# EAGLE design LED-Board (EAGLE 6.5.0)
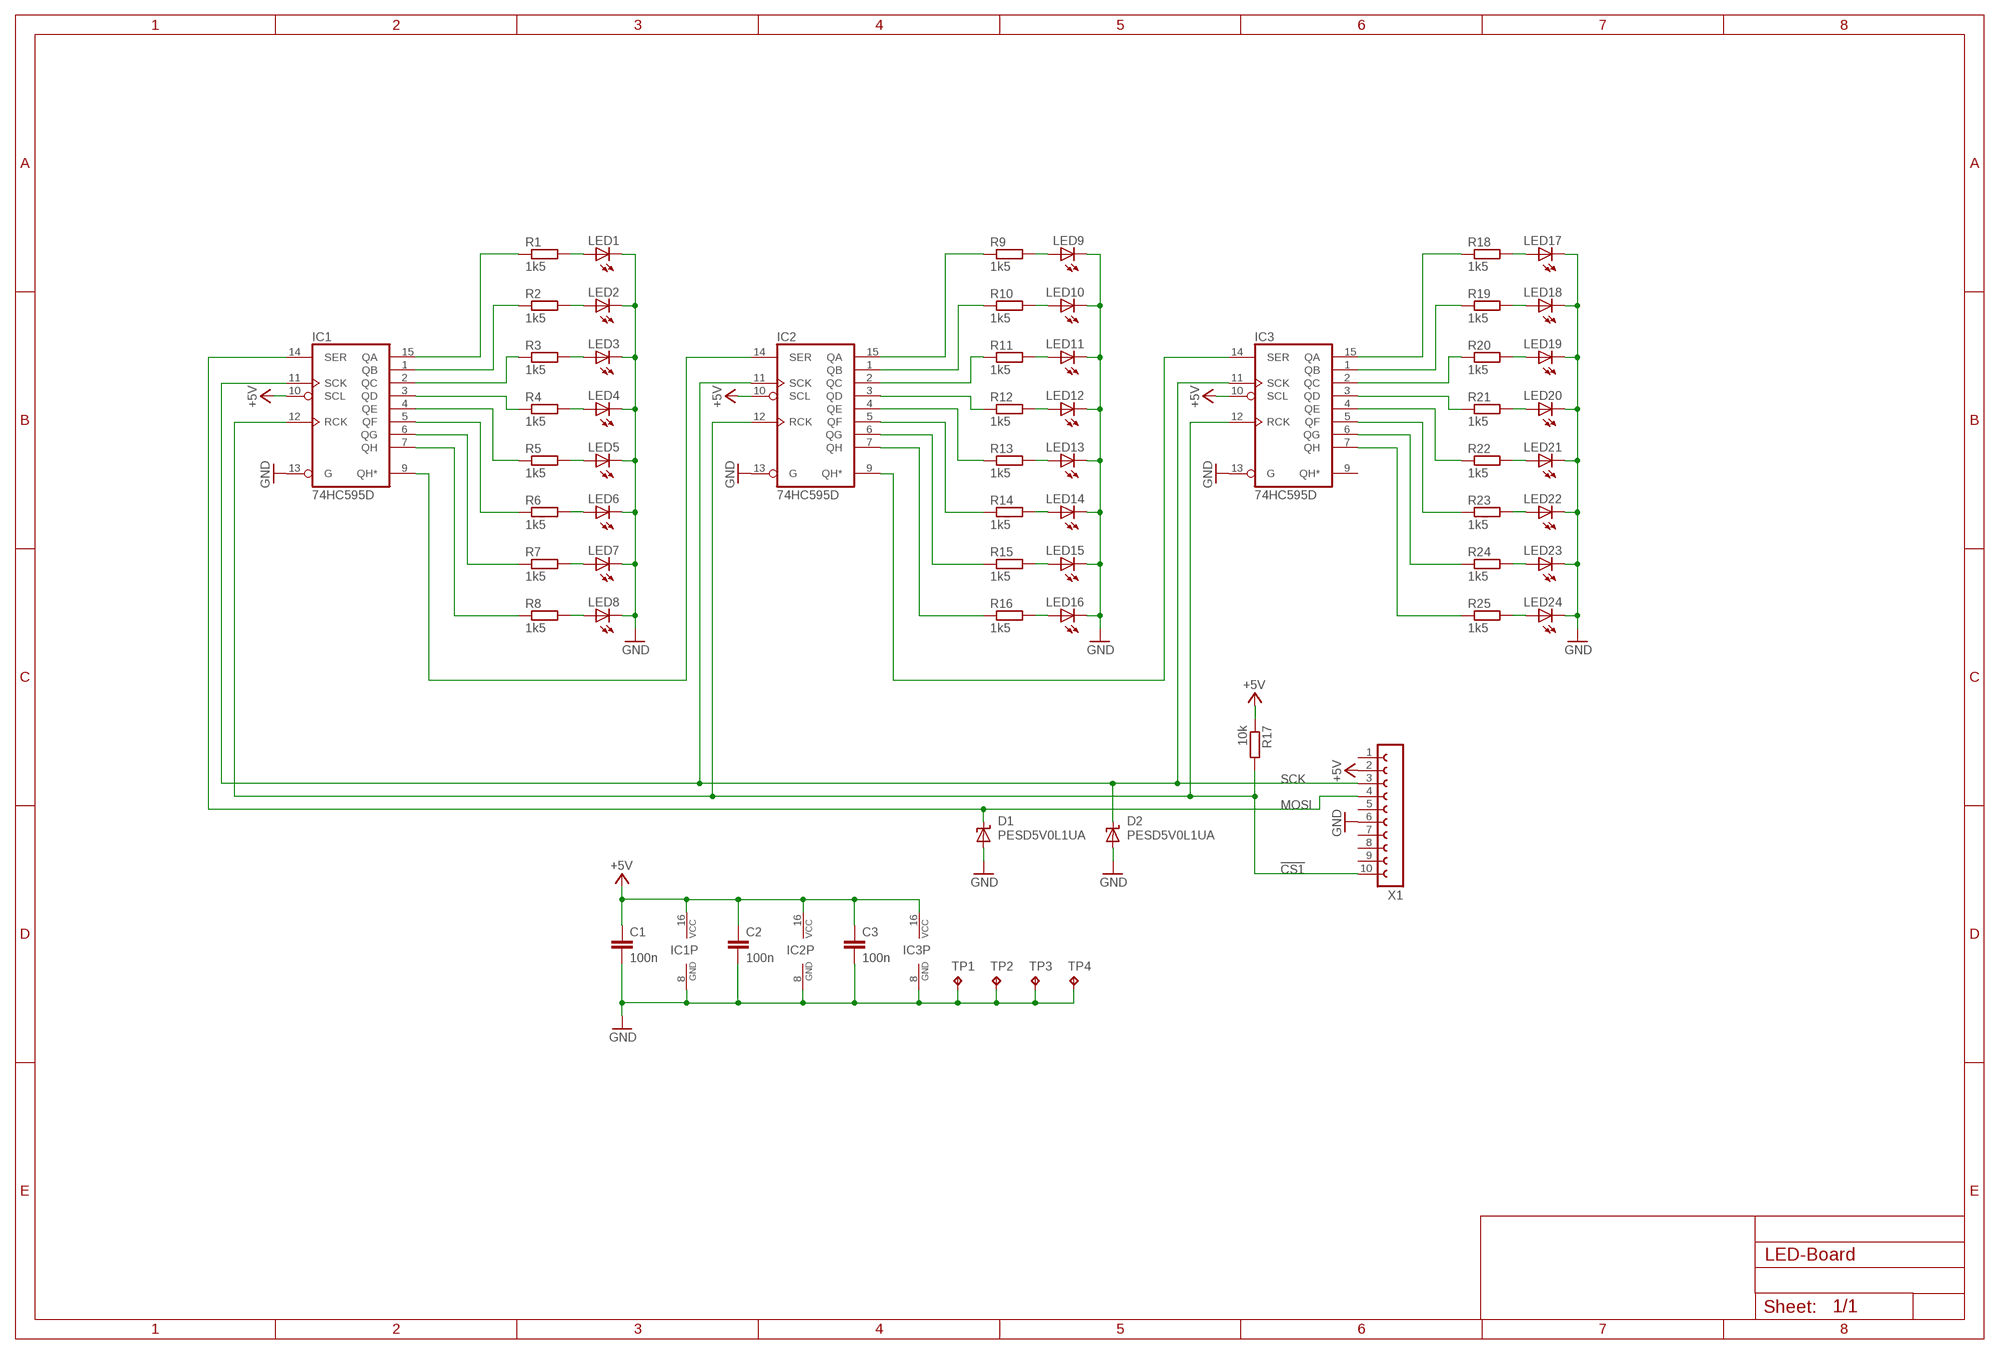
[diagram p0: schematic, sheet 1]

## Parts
C1  100n  C-EUC0603K  [C0603K]
C2  100n  C-EUC0603K  [C0603K]
C3  100n  C-EUC0603K  [C0603K]
D1  PESD5V0L1UA  SUPPRESSOR_UNI  [SOD323-W]
D2  PESD5V0L1UA  SUPPRESSOR_UNI  [SOD323-W]
IC1  74HC595D  [SO16]
IC2  74HC595D  [SO16]
IC3  74HC595D  [SO16]
LED1  LED3MM  [LED3MM]
LED2  LED3MM  [LED3MM]
LED3  LED3MM  [LED3MM]
LED4  LED3MM  [LED3MM]
LED5  LED3MM  [LED3MM]
LED6  LED3MM  [LED3MM]
LED7  LED3MM  [LED3MM]
LED8  LED3MM  [LED3MM]
LED9  LED3MM  [LED3MM]
LED10  LED3MM  [LED3MM]
LED11  LED3MM  [LED3MM]
LED12  LED3MM  [LED3MM]
LED13  LED3MM  [LED3MM]
LED14  LED3MM  [LED3MM]
LED15  LED3MM  [LED3MM]
LED16  LED3MM  [LED3MM]
LED17  LED3MM  [LED3MM]
LED18  LED3MM  [LED3MM]
LED19  LED3MM  [LED3MM]
LED20  LED3MM  [LED3MM]
LED21  LED3MM  [LED3MM]
LED22  LED3MM  [LED3MM]
LED23  LED3MM  [LED3MM]
LED24  LED3MM  [LED3MM]
R1  1k5  R-EU_R0603  [R0603]
R2  1k5  R-EU_R0603  [R0603]
R3  1k5  R-EU_R0603  [R0603]
R4  1k5  R-EU_R0603  [R0603]
R5  1k5  R-EU_R0603  [R0603]
R6  1k5  R-EU_R0603  [R0603]
R7  1k5  R-EU_R0603  [R0603]
R8  1k5  R-EU_R0603  [R0603]
R9  1k5  R-EU_R0603  [R0603]
R10  1k5  R-EU_R0603  [R0603]
R11  1k5  R-EU_R0603  [R0603]
R12  1k5  R-EU_R0603  [R0603]
R13  1k5  R-EU_R0603  [R0603]
R14  1k5  R-EU_R0603  [R0603]
R15  1k5  R-EU_R0603  [R0603]
R16  1k5  R-EU_R0603  [R0603]
R17  10k  R-EU_R0603  [R0603]
R18  1k5  R-EU_R0603  [R0603]
R19  1k5  R-EU_R0603  [R0603]
R20  1k5  R-EU_R0603  [R0603]
R21  1k5  R-EU_R0603  [R0603]
R22  1k5  R-EU_R0603  [R0603]
R23  1k5  R-EU_R0603  [R0603]
R24  1k5  R-EU_R0603  [R0603]
R25  1k5  R-EU_R0603  [R0603]
TP1  TPPAD1-13  [P1-13]
TP2  TPPAD1-13  [P1-13]
TP3  TPPAD1-13  [P1-13]
TP4  TPPAD1-13  [P1-13]
X1  MICROMATCH10SMD  [MIRCOMATCH_SMD10]

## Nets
!CS1: IC1.12(RCK) IC2.12(RCK) IC3.12(RCK) R17.2 X1.10
+5V: C1.1 C2.1 C3.1 IC1.10(SCL) IC1.16(VCC) IC2.10(SCL) IC2.16(VCC) IC3.10(SCL) IC3.16(VCC) R17.1 X1.2
GND: C1.2 C2.2 C3.2 D1.A D2.A IC1.8(GND) IC1.13(G) IC2.8(GND) IC2.13(G) IC3.8(GND) IC3.13(G) LED1.K(C) LED2.K(C) LED3.K(C) LED4.K(C) LED5.K(C) LED6.K(C) LED7.K(C) LED8.K(C) LED9.K(C) LED10.K(C) LED11.K(C) LED12.K(C) LED13.K(C) LED14.K(C) LED15.K(C) LED16.K(C) LED17.K(C) LED18.K(C) LED19.K(C) LED20.K(C) LED21.K(C) LED22.K(C) LED23.K(C) LED24.K(C) TP1.TP TP2.TP TP3.TP TP4.TP X1.6
MOSI: D1.C IC1.14(SER) X1.4
N$1: LED1.A R1.2
N$2: LED2.A R2.2
N$3: LED3.A R3.2
N$4: LED4.A R4.2
N$5: LED5.A R5.2
N$6: LED6.A R6.2
N$7: LED7.A R7.2
N$8: LED8.A R8.2
N$9: IC1.15(QA) R1.1
N$10: IC1.1(QB) R2.1
N$11: IC1.2(QC) R3.1
N$12: IC1.3(QD) R4.1
N$13: IC1.4(QE) R5.1
N$14: IC1.5(QF) R6.1
N$15: IC1.6(QG) R7.1
N$16: IC1.7(QH) R8.1
N$17: LED9.A R9.2
N$18: LED10.A R10.2
N$19: LED11.A R11.2
N$20: LED12.A R12.2
N$21: LED13.A R13.2
N$22: LED14.A R14.2
N$23: LED15.A R15.2
N$24: LED16.A R16.2
N$25: IC2.15(QA) R9.1
N$26: IC2.1(QB) R10.1
N$27: IC2.2(QC) R11.1
N$28: IC2.3(QD) R12.1
N$29: IC2.4(QE) R13.1
N$30: IC2.5(QF) R14.1
N$31: IC2.6(QG) R15.1
N$32: IC2.7(QH) R16.1
N$33: IC1.9(QH*) IC2.14(SER)
N$34: LED17.A R18.2
N$35: LED18.A R19.2
N$36: LED19.A R20.2
N$37: LED20.A R21.2
N$38: LED21.A R22.2
N$39: LED22.A R23.2
N$40: LED23.A R24.2
N$41: LED24.A R25.2
N$42: IC3.15(QA) R18.1
N$43: IC3.1(QB) R19.1
N$44: IC3.2(QC) R20.1
N$45: IC3.3(QD) R21.1
N$46: IC3.4(QE) R22.1
N$47: IC3.5(QF) R23.1
N$48: IC3.6(QG) R24.1
N$49: IC3.7(QH) R25.1
N$50: IC2.9(QH*) IC3.14(SER)
SCK: D2.C IC1.11(SCK) IC2.11(SCK) IC3.11(SCK) X1.3
Unconnected: IC3.9(QH*) X1.1 X1.5 X1.7 X1.8 X1.9

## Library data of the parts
C1-C3 = rcl:C-EU: CAPACITOR, European symbol
D1 D2 = Brunner:SUPPRESSOR_UNI
IC1-IC3 = 74xx-eu:74*595: 8-bit SHIFT REGISTER, output latch
LED1-LED24 = led:LED: LED
R1-R25 = rcl:R-EU_: RESISTOR, European symbol
TP1-TP4 = testpad:TP: Test pad
X1 = Brunner:MICROMATCH10

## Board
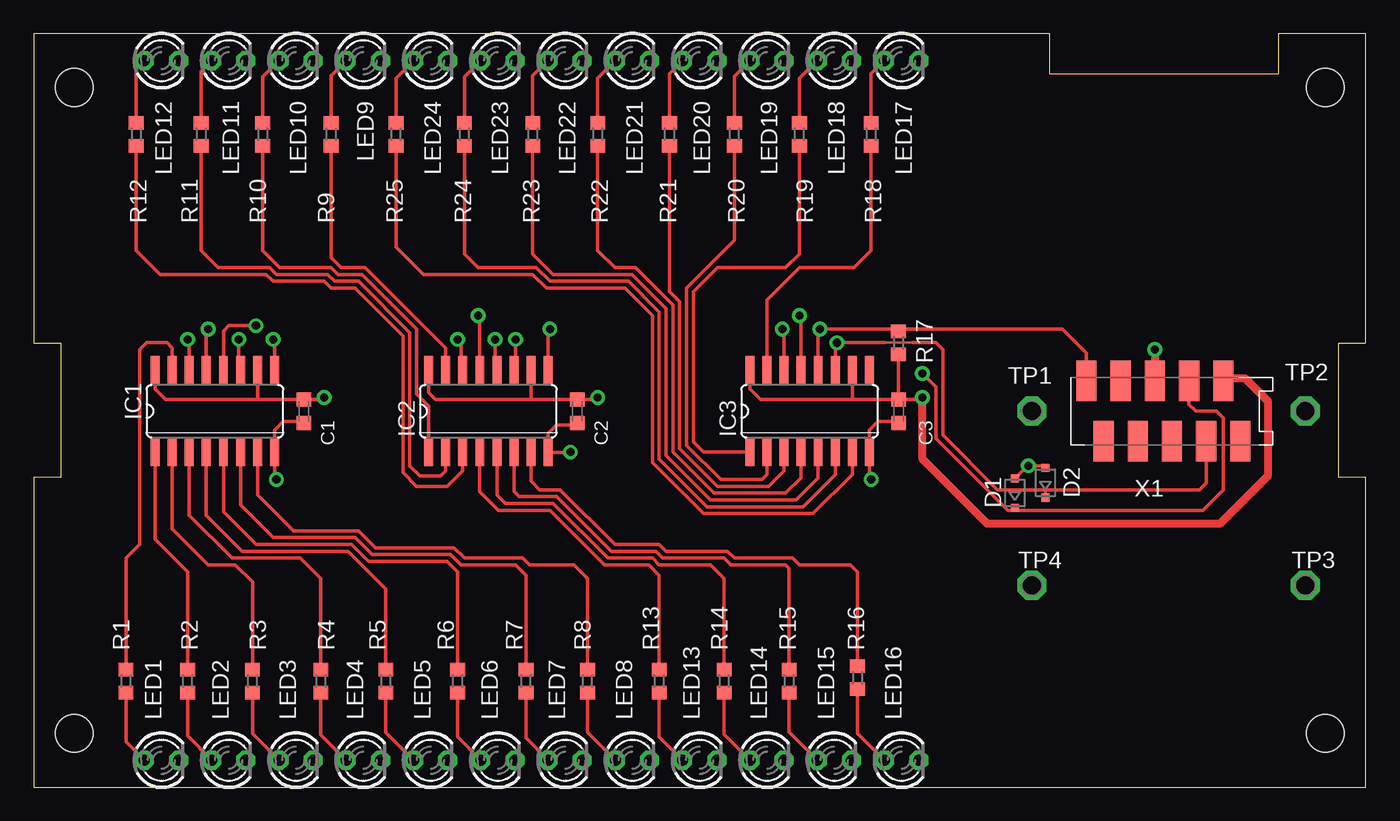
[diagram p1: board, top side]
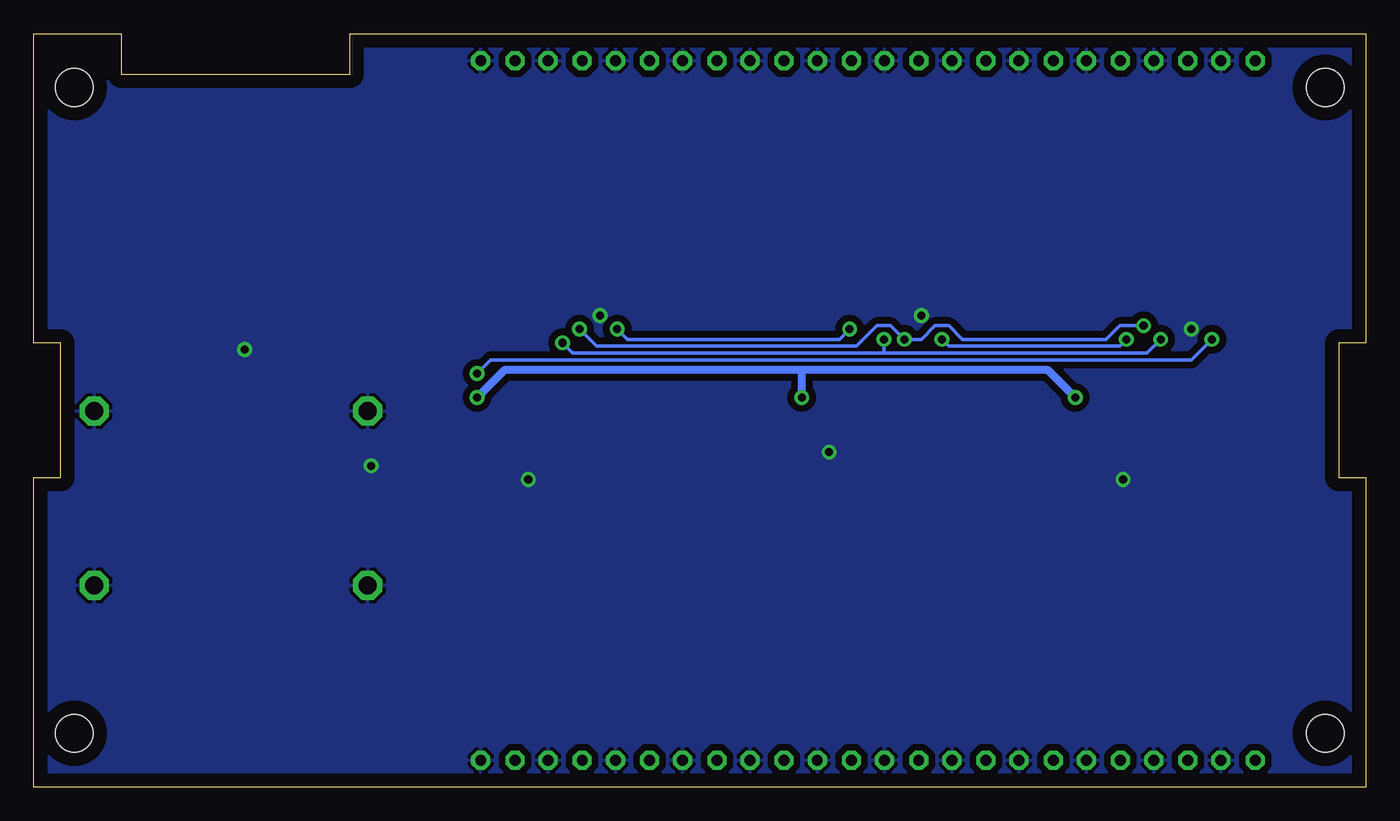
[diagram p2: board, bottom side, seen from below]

Size 99 x 56 mm. Coordinates in mm from the lower left corner, seen from the top.
Outline: 0,0 99,0 99,23 97,23 97,33 99,33 99,56 92.5,56 92.5,53 75.5,53 75.5,56 0,56 0,33 2,33 2,23 0,23 0,0
Copper layers (1*16): Top 0.035mm / dielectric 1.5mm / Bottom 0.035mm
Design rules "default *": minimum track width 10mil, minimum drill 0.6mm, track to track 0.25mm, track to pad 0.25mm, pad to pad 0.25mm, via to via 0.25mm, smd to smd 8mil, copper to edge 40mil, drill to drill 8mil, minimum pad ring 0.3mm, minimum via ring 0.25mm, stop-mask expansion 4mil, vias tented up to drill 0mil, thermal gap 10mil
Holes 2.8 mm at 3,52 3,4 96,52 96,4

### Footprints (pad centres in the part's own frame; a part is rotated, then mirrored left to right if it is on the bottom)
C0603K = smd 1.05 x 1.08: 1 -0.875,0; 2 0.875,0
SOD323-W = smd 0.6 x 0.6: A 1.1,0; C -1.1,0
SO16 = smd 0.66 x 2.032: 1 -4.445,-3.073; 2 -3.175,-3.073; 3 -1.905,-3.073; 4 -0.635,-3.073; 5 0.635,-3.073; 6 1.905,-3.073; 7 3.175,-3.073; 8 4.445,-3.073; 9 4.445,3.073; 10 3.175,3.073; 11 1.905,3.073; 12 0.635,3.073; 13 -0.635,3.073; 14 -1.905,3.073; 15 -3.175,3.073; 16 -4.445,3.073
LED3MM = drill 0.813 octagon: A -1.27,0; K 1.27,0
R0603 = smd 1 x 1.1: 1 -0.85,0; 2 0.85,0
P1-13 = drill 1.321 pad 2.159 octagon: TP 0,0
MIRCOMATCH_SMD10 = smd 1.5 x 3: 1 5.08,-2.25; 2 3.81,2.25; 3 2.54,-2.25; 4 1.27,2.25; 5 0,-2.25; 6 -1.27,2.25; 7 -2.54,-2.25; 8 -3.81,2.25; 9 -5.08,-2.25; 10 -6.35,2.25

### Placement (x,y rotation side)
C1  20.07,27.94 270 top
C2  40.39,27.94 270 top
C3  64.27,27.94 270 top
D1  72.91,21.84 90 top
D2  75.19,22.61 90 top
IC1  13.47,27.94 0 top
IC2  33.79,27.94 0 top
IC3  57.67,27.94 0 top
LED1  9.5,2 0 top
LED2  14.5,2 0 top
LED3  19.5,2 0 top
LED4  24.5,2 0 top
LED5  29.5,2 0 top
LED6  34.5,2 0 top
LED7  39.5,2 0 top
LED8  44.5,2 0 top
LED9  24.5,54 0 top
LED10  19.5,54 0 top
LED11  14.5,54 0 top
LED12  9.5,54 0 top
LED13  49.5,2 0 top
LED14  54.5,2 0 top
LED15  59.5,2 0 top
LED16  64.5,2 0 top
LED17  64.5,54 0 top
LED18  59.5,54 0 top
LED19  54.5,54 0 top
LED20  49.5,54 0 top
LED21  44.5,54 0 top
LED22  39.5,54 0 top
LED23  34.5,54 0 top
LED24  29.5,54 0 top
R1  6.87,7.87 270 top
R2  11.44,7.87 270 top
R3  16.26,7.87 270 top
R4  21.34,7.87 270 top
R5  26.17,7.87 270 top
R6  31.5,7.87 270 top
R7  36.58,7.87 270 top
R8  41.16,7.87 270 top
R9  22.11,48.51 90 top
R10  17.03,48.51 90 top
R11  12.45,48.51 90 top
R12  7.63,48.51 90 top
R13  46.49,7.87 270 top
R14  51.32,7.87 270 top
R15  56.14,7.87 270 top
R16  61.22,8.13 270 top
R17  64.27,33.02 90 top
R18  62.24,48.51 90 top
R19  56.9,48.51 90 top
R20  52.08,48.51 90 top
R21  47.25,48.51 90 top
R22  41.92,48.51 90 top
R23  37.09,48.51 90 top
R24  32.01,48.51 90 top
R25  26.93,48.51 90 top
TP1  74.18,27.94 0 top
TP2  94.5,27.94 0 top
TP3  94.5,14.99 0 top
TP4  74.18,14.99 0 top
U$1  [A4L-LOC]  not placed on the board
X1  84.59,27.94 0 top

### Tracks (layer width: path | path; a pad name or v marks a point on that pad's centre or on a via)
!CS1  (via drill 0.6)
  Top 0.254: v16.52,34.29 14.49,34.29 14.11,33.91 IC1.12 | 34.55,30.99 34.53,31.01 IC2.12 34.3,31.14 v34.3,33.27 | IC3.12 58.3,33.91 v58.43,34.04 64.1,34.04 R17.2 64.44,34.04 76.46,34.04 78.24,32.26 X1.10 78.24,30.16
  Bottom 0.254: v16.52,34.29 18.3,34.29 19.31,33.27 29.98,33.27 31,34.29 32.01,34.29 33.03,33.27 v34.3,33.27 35.31,34.29 36.33,34.29 37.85,32.77 57.16,32.77 v58.43,34.04
+5V  (via drill 0.6)
  Top 0.254: IC1.16 9.03,29.59 9.8,28.82 16.52,28.82 | 16.52,28.82 C1.1 21.46,28.82 v21.6,28.96 | 36.84,28.82 C2.1 41.78,28.82 v41.92,28.96 | 36.84,28.82 29.87,28.82 29.34,29.34 IC2.16 | IC2.10 36.97,28.94 36.84,28.82 | C3.1 60.97,28.82 | 60.97,28.82 54,28.82 53.22,29.59 IC3.16 | IC3.10 60.84,28.94 60.97,28.82 | IC1.10 16.64,28.94 16.52,28.82 | R17.1 C3.1 | C3.1 65.91,28.82 v66.05,28.96
  Top 0.61: v66.05,28.96 66.05,24.38 70.87,19.56 88.15,19.56 91.7,23.11 91.7,28.7 90.03,30.38 88.59,30.38 X1.2
  Bottom 0.61: v21.6,28.96 23.63,30.99 41.92,30.99 | v41.92,28.96 41.92,30.99 | 41.92,30.99 64.02,30.99 v66.05,28.96
GND  (via drill 0.6)
  Top 0.254: IC1.8 17.91,26.54 18.55,27.18 19.96,27.18 C1.2 | IC1.8 17.91,24.77 | C2.2 40.25,26.92 38.87,26.92 38.23,26.29 IC2.8 39.89,24.87 v39.89,24.89 | IC2.13 33.16,34.92 v33.03,35.05 | IC3.13 57.03,34.92 v56.9,35.05 | IC1.13 12.84,33.91 v12.96,34.04 | IC1.8 17.91,22.99 v18.04,22.86 | v62.24,22.86 62.11,22.99 IC3.8 62.11,26.54 62.75,27.18 64.16,27.18 C3.2 | D2.A 75.19,23.88 v73.92,23.88 73.84,23.88 D1.A
  Top 0.61: v83.32,32.51 X1.6
  pour Bottom (isolate 0.5): -0.25,57.66 99.58,57.66 99.58,0 0,0 0,39.88
MOSI  (via drill 0.6)
  Top 0.254: IC1.14 11.56,33.15 v11.44,33.27 | 72.91,20.57 86.88,20.57 88.4,22.1 88.4,27.43 87.89,27.94 86.37,27.94 85.86,28.45 X1.4 | 72.91,20.57 72.4,20.57 67.06,25.91 67.06,29.72 v66.05,30.73 | D1.C 72.91,20.57
  Bottom 0.254: v11.44,33.27 12.96,31.75 65.03,31.75 v66.05,30.73
N$1
  Top 0.254: R1.2 6.87,3.36 LED1.A
N$2
  Top 0.254: R2.2 11.44,3.79 LED2.A
N$3
  Top 0.254: R3.2 16.26,3.97 LED3.A
N$4
  Top 0.254: R4.2 21.34,3.89 LED4.A
N$5
  Top 0.254: R5.2 26.17,4.06 LED5.A
N$6
  Top 0.254: R6.2 31.5,3.73 LED6.A
N$7
  Top 0.254: R7.2 36.58,3.65 LED7.A
N$8
  Top 0.254: R8.2 41.16,4.07 LED8.A
N$9
  Top 0.254: IC1.15 10.29,32.64 9.91,33.02 8.39,33.02 7.88,32.51 7.88,18.03 6.87,17.02 R1.1
N$10
  Top 0.254: IC1.1 9.03,18.41 11.44,16 R2.1
N$11
  Top 0.254: IC1.2 10.29,19.18 12.96,16.51 14.99,16.51 16.26,15.24 R3.1
N$12
  Top 0.254: IC1.3 11.56,20.19 14.74,17.02 19.82,17.02 21.34,15.49 R4.1
N$13
  Top 0.254: IC1.4 12.84,20.19 15.5,17.53 23.38,17.53 26.17,14.73 R5.1
N$14
  Top 0.254: IC1.5 14.11,20.45 16.52,18.03 23.63,18.03 24.9,16.76 30.74,16.76 31.5,16 R6.1
N$15
  Top 0.254: IC1.6 15.38,20.95 17.79,18.54 23.88,18.54 25.15,17.27 31,17.27 31.76,16.51 35.82,16.51 36.58,15.75 R7.1
N$16
  Top 0.254: IC1.7 16.64,21.72 19.31,19.05 24.14,19.05 25.41,17.78 31.25,17.78 32.01,17.02 36.33,17.02 36.84,16.51 40.14,16.51 41.16,15.49 R8.1
N$17
  Top 0.254: R9.2 22.11,52.88 LED9.A
N$18
  Top 0.254: R10.2 17.03,52.8 LED10.A
N$19
  Top 0.254: R11.2 12.45,53.22 LED11.A
N$20
  Top 0.254: R12.2 7.63,53.4 LED12.A
N$21
  Top 0.254: R13.2 46.49,3.74 LED13.A
N$22
  Top 0.254: R14.2 51.32,3.91 LED14.A
N$23
  Top 0.254: R15.2 56.14,4.09 LED15.A
N$24
  Top 0.254: R16.2 61.22,4.01 LED16.A
N$25
  Top 0.254: IC2.15 30.61,32.64 24.65,38.61 22.87,38.61 22.11,39.37 R9.1
N$26
  Top 0.254: IC2.1 29.34,28.32 28.46,29.21 28.46,34.04 24.39,38.1 22.61,38.1 22.11,38.61 18.3,38.61 17.03,39.88 R10.1
N$27
  Top 0.254: IC2.2 30.61,23.5 30.23,23.11 28.71,23.11 27.95,23.88 27.95,33.78 24.14,37.59 22.36,37.59 21.85,38.1 18.04,38.1 17.53,38.61 13.72,38.61 12.45,39.88 R11.1
N$28
  Top 0.254: IC2.3 31.88,23.5 30.74,22.35 28.46,22.35 27.44,23.37 27.44,33.53 23.88,37.08 22.11,37.08 21.6,37.59 17.79,37.59 17.28,38.1 9.41,38.1 7.63,39.88 R12.1
N$29
  Top 0.254: IC2.4 33.16,21.97 34.55,20.57 38.36,20.57 42.43,16.51 45.73,16.51 46.49,15.75 R13.1
N$30
  Top 0.254: IC2.5 34.42,21.72 35.06,21.08 38.62,21.08 42.68,17.02 45.98,17.02 46.49,16.51 50.3,16.51 51.32,15.49 R14.1
N$31
  Top 0.254: IC2.6 35.7,21.97 36.08,21.59 38.87,21.59 42.93,17.53 46.24,17.53 46.74,17.02 51.32,17.02 51.82,16.51 55.89,16.51 56.14,16.26 R15.1
N$32
  Top 0.254: IC2.7 36.97,22.73 37.6,22.1 39.12,22.1 43.19,18.03 46.49,18.03 47,17.53 51.57,17.53 52.08,17.02 56.4,17.02 56.9,16.51 60.71,16.51 61.22,16 R16.1
N$33  (via drill 0.6)
  Top 0.254: v31.5,33.27 31.76,33.02 31.76,31.14 IC2.14 | IC1.9 17.91,33.15 v17.79,33.27
  Bottom 0.254: v17.79,33.27 18.3,32.77 31,32.77 v31.5,33.27 31.76,33.02
N$34
  Top 0.254: R18.2 62.24,53.01 LED17.A
N$35
  Top 0.254: R19.2 56.9,52.67 LED18.A
N$36
  Top 0.254: R20.2 52.08,52.85 LED19.A
N$37
  Top 0.254: R21.2 47.25,53.02 LED20.A
N$38
  Top 0.254: R22.2 41.92,52.69 LED21.A
N$39
  Top 0.254: R23.2 37.09,52.86 LED22.A
N$40
  Top 0.254: R24.2 32.01,52.78 LED23.A
N$41
  Top 0.254: R25.2 26.93,52.7 LED24.A
N$42
  Top 0.254: IC3.15 54.49,36.2 56.9,38.61 60.97,38.61 62.24,39.88 R18.1
N$43
  Top 0.254: IC3.1 53.2,24.89 49.79,24.89 49.03,25.65 49.03,36.83 50.81,38.61 55.89,38.61 56.9,39.62 R19.1
N$44
  Top 0.254: IC3.2 54.49,23.24 54.11,22.86 51.06,22.86 48.52,25.4 48.52,37.08 52.08,40.64 R20.1
N$45
  Top 0.254: IC3.3 55.76,23.5 54.62,22.35 50.81,22.35 48.01,25.15 48.01,36.07 47.25,36.83 R21.1
N$46
  Top 0.254: IC3.4 57.03,22.99 55.89,21.84 50.55,21.84 47.51,24.89 47.51,35.81 44.71,38.61 43.19,38.61 41.92,39.88 R22.1
N$47
  Top 0.254: IC3.5 58.3,22.99 56.65,21.34 50.3,21.34 47,24.64 47,35.56 44.46,38.1 38.62,38.1 37.09,39.62 R23.1
N$48
  Top 0.254: IC3.6 59.57,23.24 57.16,20.83 50.05,20.83 46.49,24.38 46.49,35.31 44.2,37.59 38.36,37.59 37.35,38.61 33.03,38.61 32.01,39.62 R24.1
N$49
  Top 0.254: IC3.7 60.84,23.24 57.92,20.32 49.79,20.32 45.98,24.13 45.98,35.05 43.95,37.08 38.11,37.08 37.09,38.1 28.96,38.1 26.93,40.13 R25.1
N$50  (via drill 0.6)
  Top 0.254: IC2.9 38.23,33.91 v38.36,34.04 | IC3.14 55.76,33.91 v55.63,34.04
  Bottom 0.254: v38.36,34.04 39.12,33.27 54.87,33.27 v55.63,34.04
SCK  (via drill 0.6)
  Top 0.2: 63.25,33.02 65.29,33.02
  Top 0.254: IC1.11 15.38,31.11 15.25,31.24 v15.25,33.27 | v35.82,33.27 35.82,31.14 IC2.11 | IC3.11 59.57,32.89 v59.7,33.02 63.25,33.02 | 75.19,22.1 86.62,22.1 87.13,22.61 X1.3 | 75.19,22.1 71.64,22.1 67.57,26.16 67.57,32.51 67.06,33.02 65.29,33.02 | D2.C 75.19,22.1
  Bottom 0.254: v15.25,33.27 16.26,32.26 35.82,32.26 | 35.82,32.26 58.94,32.26 v59.7,33.02 | 35.82,32.26 v35.82,33.27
